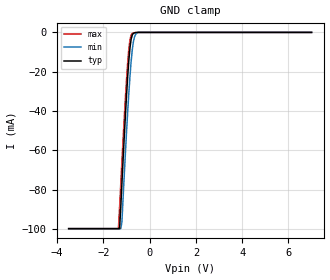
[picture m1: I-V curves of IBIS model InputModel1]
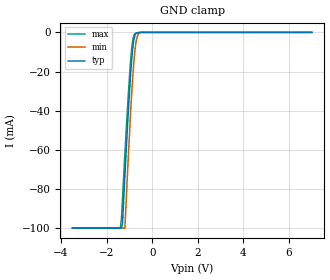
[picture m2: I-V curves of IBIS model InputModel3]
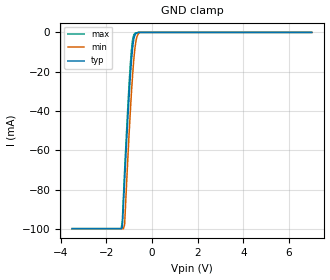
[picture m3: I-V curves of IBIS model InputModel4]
[IBIS Ver]   2.1
[File name]   e_016xd3.ibs   | e_= TSOP, f016xd= abbr chip name, 3=3.3V Vcc
[File Rev]   2.40
[Date]   13-February-96
[Source]   File generated from lab measurements at Intel Corporation
[Notes]   Rev 2.00 fixes simulation model flaw.
   Rev 2.01 fixes typo errors in comments only.
   Rev 2.10 adds two omitted comment markers (|) to InputModel1
   and implements improvements for Quad parser IBIS2XTK:
   * adds zero current [POWER_clamp] to input models
   * changes model name from "I/O" to "InputOutput"
   * changes model type "Open_Drain" to "Open_drain"
   Rev 2.20 adds required dV/dt_r for OpenDrainOutput.
   Rev 2.30 adds 3/5# pin to pin #1.  The input model remains the
   same as it was included in rev 2.20, though the pin
   was a no connect in that model.
   Rev 2.40 All data was replaced by actual measurements
   performed in a lab.
[Disclaimer] INTEL DEVELOPER'S SOFTWARE LICENSE AGREEMENT
| BY USING THIS SOFTWARE, YOU ARE AGREEING TO BE BOUND
| BY THE TERMS OFTHIS AGREEMENT.  DO NOT USE THE SOFTWARE
| UNTIL YOU HAVE CAREFULLY READAND AGREED TO THE FOLLOWING
| TERMS AND CONDITIONS.  IF YOU DO NOT AGREETO THE TERMS
| OF THIS AGREEMENT, PROMPTLY RETURN THE SOFTWARE PACKAGE
| ANDANY ACCOMPANYING ITEMS.
| IF YOU USE THIS SOFTWARE, YOU WILL BE BOUND BY THE TERMS
| OF THIS AGREEMENT
| LICENSE: Intel Corporation ("Intel") grants you the non-exclusive right
| to use the enclosed software program ("Software").  You will not use,
| copy, modify, rent, sell or transfer the Software or any portion
| thereof, except as provided in this Agreement.
| System OEM Developers may:
| 1.   Copy the Software for support, backup or archival purposes;
| 2.   Install, use, or distribute Intel owned Software in object code
|   only;
| 3.   Modify and/or use Software source code that Intel directly makes
|   available to you as an OEM Developer;
| 4.   Install, use, modify, distribute, and/or make or have made
|   derivatives ("Derivatives") of Intel owned Software under the
|   terms and conditions in this Agreement, ONLY if you are a System
|   OEM Developer and NOT an end-user.
| RESTRICTIONS:
| YOU WILL NOT:
| 1.   Copy the Software, in whole or in part, except as provided for
|   in this Agreement;
| 2.   Decompile or reverse engineer any Software provided in object
|   code format;
| 3.   Distribute any Software or Derivative code to any end-users,
|   unless approved by Intel in a prior writing.
| TRANSFER: You may transfer the Software to another OEM
| Developer if thereceiving party agrees to the terms of this
| Agreement at the sole risk of any receiving party.
| OWNERSHIP AND COPYRIGHT OF SOFTWARE:
| Title to the Software and all copies thereof remain with Intel
| or its vendors.  The Software iscopyrighted and is protected by
| United States and international copyright laws.  You will not
| remove the copyright notice from the Software.  You agree to
| prevent any unauthorized copying of the Software.
| DERIVATIVE WORK: OEM Developers that make or have made
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[Copyright]   Copyright 1995,1996, Intel Corporation, All Rights Reserved
[Component]   E28F016XD   | 56-lead TSOP package, 28F016XD
[Manufacturer]  Intel   | DRAM-Interface Flash Memory
|   | operating in 3.3V Vcc range
[Package]
|The following values apply for the Copper leadframe.
|Variable   typ   min   max
  R_pkg   48m   41m   54m
  L_pkg   4.92nH   4.44nH   5.39nH
  C_pkg   0.48pF   0.45pF   0.50pF
|The following values apply for the Alloy-42 leadframe.
| R_pkg   195m   180m   210m
| L_pkg   4.92nH   4.44nH   5.39nH
| C_pkg   0.48pF   0.45pF   0.50pF
|******************Pin Defintions*************************************
[Pin] signal_name   model_name   R_pin   L_pin   C_pin
  1   3/5#   InputModel1
  2   GND   InputModel1
  3   NC   InputModel2
  4   A9   InputModel3
  5   A8   InputModel3
  6   A7   InputModel1
  7   A6   InputModel1
  8   A5   InputModel1
  9   VCC   POWER
 10   RAS#   InputModel1
 11   CAS#   InputModel3
 12   NC   InputModel1
 13   NC   InputModel1
 14   GND   InputModel1
 15   VPP   POWER
 16   RP#   InputModel4
 17   NC   InputModel1
 18   NC   InputModel1
 19   NC   InputModel1
 20   NC   InputModel1
 21   GND   GND
 22   NC   InputModel1
 23   NC   InputModel1
 24   A4   InputModel1
 25   A3   InputModel1
 26   A2   InputModel1
 27   A1   InputModel1
 28   A0   InputModel1
 29   NC   InputModel5
 30   NC   InputModel5
 31   VCC   InputModel1
 32   NC   InputModel1
 33   DQ0   InputOutput
 34   DQ8   InputOutput
 35   DQ1   InputOutput
 36   DQ9   InputOutput
 37   VCC   POWER
 38   DQ2   InputOutput
 39   DQ10   InputOutput
 40   DQ3   InputOutput
 41   DQ11   InputOutput
 42   GND   GND
 43   VCC   POWER
 44   DQ4   InputOutput
 45   DQ12   InputOutput
 46   DQ5   InputOutput
 47   DQ13   InputOutput
 48   GND   GND
 49   DQ6   InputOutput
 50   DQ14   InputOutput
 51   DQ7   InputOutput
 52   DQ15   InputOutput
 53   RY/BY#   OpenDrainOutput
 54   OE#   InputModel1
 55   WE#   InputModel4
 56   WP#   InputModel1
|*******************Input Model 2**********************************
[Model]   InputModel2
Model_type   Input
|   for pin3(NC)
Vinl = 0.8V
Vinh = 2.0V
|Variable   typ   min   max
C_comp   5.61p   NA   7.6p
[Voltage Range]   3.3V   3.0V   3.6V
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| Models and submodels in the file (7): InputModel1 (Input), InputModel2 (Input), InputModel3 (Input), InputModel4 (Input), InputModel5 (Input), InputOutput (I/O), OpenDrainOutput (Open_drain)
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|**********************Input Model 1*************************************
[Model]   InputModel1
Model_type   Input
|   Model for pin1(3/5#), pin2(GND), pin12(NC), pin13(NC),
|   pin14(GND), pin17(NC), pin18(NC), pin19(NC), pin20(NC),
|   pin22(NC), pin23(NC), pin31(VCC), pin32(NC), OE#, WP#,
|   A[7:0], and RAS#.
Vinl = 0.8V
Vinh = 2.0V
|Variable   typ   min   max
C_comp   5.61p   NA   7.6p
[Voltage Range]   3.3V   3.0V   3.6V
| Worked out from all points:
|   GND clamp passes 1 mA (typ) near -0.73 V on its own axis
[GND_clamp]
|Voltage I(typ)   I(min)   I(max)
-3.5V     -99.85mA   -99.84mA   -99.84mA
-1.35V    -99.85mA   -99.84mA   -99.84mA
-1.3V     -99.85mA   -99.84mA   -89.12mA
-1.25V    -89.22mA   -99.84mA   -77.38mA
-1.2V     -77.08mA   -96.6mA    -65.98mA
-1.05V    -42.59mA   -61.78mA   -33.74mA
-950mV    -22.54mA   -40.48mA   -15.51mA
-850mV    -7.789mA   -22.25mA   -3.733mA
-750mV    -1.271mA   -8.689mA   -470.3uA
-650mV    -204.5uA   -2.102mA   -138.8uA
-500mV    0A         0A         0A
7V        0A         0A         0A
[POWER_clamp]
| Input buffer circuits of this product do not intrinsically
| require a [POWER_clamp] definition.  This zero current
| [POWER_clamp] is provided for compatibility with some ibis
| parsers.
|Voltage  I(typ)   I(min)   I(max)
-3.3V     0A         0A         0A
-3V       0A         0A         0A
6.3V      0A         0A         0A
6.6V      0A         0A         0A
|*********************Input Model 3*****************************************
[Model]   InputModel3
Model_type   Input
|   for A[9], A[8], CAS#
Vinl = 0.8V
Vinh = 2.0V
|Variable   typ   min   max
C_comp   5.61p   NA   7.6p
[Voltage Range]   3.3V   3.0V   3.6V
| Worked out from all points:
|   GND clamp passes 1 mA (typ) near -0.73 V on its own axis
[GND_clamp]
|Voltage I(typ)   I(min)   I(max)
-3.5V     -99.85mA   -99.84mA   -99.85mA
-1.4V     -99.85mA   -99.84mA   -99.85mA
-1.35V    -99.85mA   -99.84mA   -95.24mA
-1.3V     -97.13mA   -99.84mA   -84.18mA
-1.2V     -73.73mA   -99.84mA   -62.47mA
-1.05V    -40.94mA   -63.77mA   -32.1mA
-950mV    -21.84mA   -41.27mA   -14.87mA
-850mV    -7.699mA   -22.19mA   -3.685mA
-750mV    -1.334mA   -8.361mA   -527.4uA
-650mV    -247.7uA   -1.963mA   -174.6uA
-500mV    0A         0A         0A
7V        0A         0A         0A
[POWER_clamp]
| Input buffer circuits of this product do not intrinsically
| require a [POWER_clamp] definition.  This zero current
| [POWER_clamp] is provided for compatibility with some ibis
| parsers.
|Voltage  I(typ)   I(min)   I(max)
-3.3V     0A         0A         0A
-3V       0A         0A         0A
6.3V      0A         0A         0A
6.6V      0A         0A         0A
|*********************Input Model 4****************************************
[Model]   InputModel4
Model_type   Input
|   for RP#, WE#
Vinl = 0.8V
Vinh = 2.0V
| Variable   typ   min   max
C_comp   5.61p   NA   7.6p
[Voltage Range]   3.3V   3.0V   3.6V
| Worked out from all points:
|   GND clamp passes 1 mA (typ) near -0.73 V on its own axis
[GND_clamp]
|Voltage I(typ)   I(min)   I(max)
-3.5V     -99.85mA   -99.85mA   -99.84mA
-1.35V    -99.85mA   -99.85mA   -99.84mA
-1.3V     -99.17mA   -99.85mA   -95.89mA
-1.2V     -75.42mA   -97.77mA   -70.17mA
-1.05V    -41.92mA   -61.97mA   -35.8mA
-950mV    -22.4mA    -40.13mA   -16.24mA
-900mV    -14.28mA   -30.3mA    -8.781mA
-850mV    -7.903mA   -21.6mA    -3.827mA
-750mV    -1.346mA   -8.101mA   -477.5uA
-650mV    -214.7uA   -1.881mA   -139.1uA
-550mV    0A         0A         0A
7V        0A         0A         0A
[POWER_clamp]
| Input buffer circuits of this product do not intrinsically
| require a [POWER_clamp] definition.  This zero current
| [POWER_clamp] is provided for compatibility with some ibis
| parsers.
|Voltage  I(typ)   I(min)   I(max)
-3.3V     0A         0A         0A
-3V       0A         0A         0A
6.3V      0A         0A         0A
6.6V      0A         0A         0A
